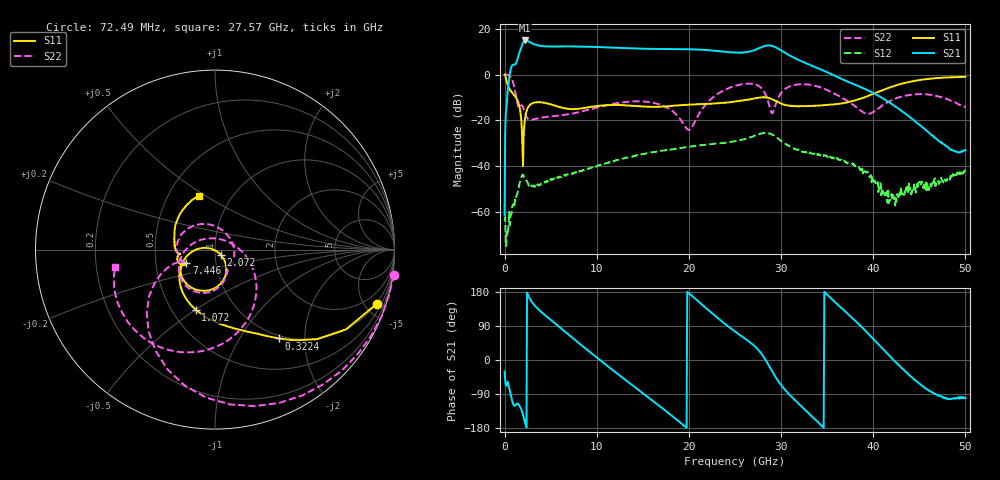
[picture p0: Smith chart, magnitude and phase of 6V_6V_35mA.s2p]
! MARKI MICROWAVE INC.
! Date:  1/07/2020
! Model Number:  APM-6849CH
! Description:  2-port Small Signal S-parameter data for APM-6849CH
! Frequency Range:  10 MHz to 50 GHz
! Port Configuration:  PORT 1: Input
!  PORT 2: Output
! Bias Condition: Vc = +6V, Vb = +6V
! APM-6849CH s2p files are only valid for small signal conditions (below -5 dBm input power)
!S2P File: Measurements: Mag<S11> Ang<S11>, Mag<S21> Ang<S21>, Mag<S12> Ang<S12>, Mag<S22> Ang<S22>!row 1
# Hz S  dB  R 50
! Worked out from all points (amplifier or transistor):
!   801 points, 10 MHz to 50 GHz, reference 50 ohm
!   highest |S21| = 14.9 dB at 2.26 GHz (marker M1)
!   |S21| within 3 dB of that: 1.822 GHz to 10.96 GHz (9.141 GHz wide, 143 % of centre)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
!   unconditionally stable (mu >= 1): 198.2 MHz to end of sweep
!   at 8.321 GHz: K = 14.67, MAG = 12.5 dB, |S12| = -42.1 dB
!   at 25 GHz: K = 3.03, MAG = 11.6 dB, |S12| = -29.1 dB
!   at 50 GHz: K = 511.22, MAG = -25.8 dB, |S12| = -41.6 dB
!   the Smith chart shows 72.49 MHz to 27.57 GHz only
!   S11 on the Smith chart (normalised r, x): 72.49 MHz: 0.95, -6.02; 322.4 MHz: 0.95, -1.50; 1.072 GHz: 0.65, -0.50; 2.072 GHz: 1.06, -0.06; 7.446 GHz: 0.72, -0.11; 27.57 GHz: 0.71, +0.47
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1e7  0.00 -2.8  -61.53 -30.3  -63.43 56.2  0.07 -1.1
7.24875e7  -0.43 -18.4  -25.19 -52.6  -62.36 33.7  0.06 -8.0
3.224375e8  -4.30 -54.3  -8.06 -57.2  -70.13 63.6  -0.12 -36.3
1.072288e9  -9.07 -107.8  4.32 -120.8  -57.95 -51.7  -5.71 -137.2
2.072088e9  -27.38 -41.2  14.37 -150.8  -44.24 -134.6  -14.99 130.6
2.25955e9  -18.37 -58.3  14.90 -168.1  -45.77 -151.9  -17.24 96.4
2.821938e9  -13.02 -94.9  13.96 158.6  -48.87 -166.7  -19.76 27.3
3.696762e9  -12.08 -125.3  12.68 133.2  -48.09 -168.9  -19.05 -15.2
7.446012e9  -15.11 -154.8  12.29 57.0  -43.21 147.8  -17.00 -61.2
8.383325e9  -14.74 -152.8  12.25 38.2  -42.19 139.9  -16.12 -66.4
1.063288e10  -13.49 -158.4  11.95 -5.7  -39.17 112.7  -13.81 -82.2
1.313238e10  -13.44 -169.2  11.54 -52.9  -36.38 81.4  -11.99 -106.5
1.669416e10  -14.10 -173.1  11.16 -119.1  -33.43 32.9  -12.88 -153.0
2.038092e10  -13.11 178.4  10.99 168.3  -31.33 -22.7  -22.60 43.4
2.269296e10  -12.67 166.8  10.45 119.7  -30.27 -63.0  -9.69 -45.3
2.5005e10  -11.78 149.2  9.59 75.1  -29.09 -105.5  -4.95 -96.0
2.756699e10  -10.16 106.6  11.42 25.6  -26.10 -170.9  -4.95 -170.1
2.862928e10  -10.18 74.8  12.73 -12.4  -25.70 146.5  -12.22 117.7
2.975405e10  -12.19 45.3  11.15 -57.7  -28.22 100.9  -9.70 -56.2
3.337832e10  -13.68 -4.8  3.75 -149.4  -34.64 29.4  -4.63 -158.8
4.168916e10  -5.81 -37.6  -12.01 12.9  -56.08 107.6  -11.87 -153.4
5e10  -0.96 -97.8  -33.01 -100.6  -41.56 -65.0  -14.20 109.0
